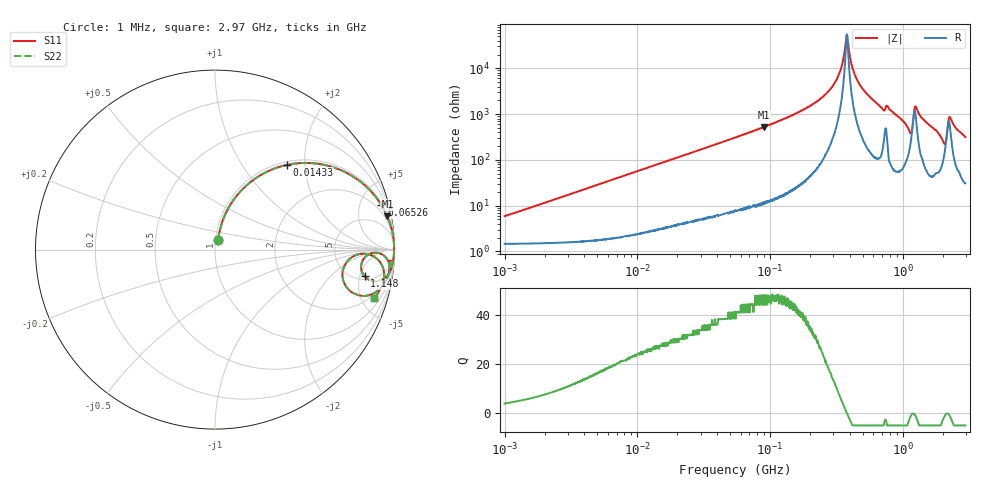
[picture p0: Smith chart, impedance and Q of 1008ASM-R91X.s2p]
!s-Parameter Generated by FASTRON Sdn. Bhd.
!FASTRON P/N : 1008ASM-R91X
!Keysight Technologies: E4991B_MY54100416_A.01.15
!Date: Tue Nov 21 09:40:02 2023
!Version  :Rev00  Wed Nov 22 15:18:00 2023
!Data & Calibration Information:
!Freq  S11  S21  S12  S22
!PortZ  Port1:50+j0  Port2:50+j0
!When reading reference impedance value at option line is always used.
! Remarks : This data is being provided solely for informational purposes.
# Hz S dB R 50
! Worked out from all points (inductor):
!   1599 points, 1 MHz to 2.97 GHz, reference 50 ohm
!   read as one part in series: L = 911 nH near 1.036 MHz
!   highest Q = 47.7 at 89.44 MHz (marker M1), where L = 924 nH
!   self-resonance near 377.9 MHz
!   S11 on the Smith chart (normalised r, x): 1 MHz: 1.03, +0.11; 14.33 MHz: 1.06, +1.61; 65.26 MHz: 1.18, +7.41; 1.148 GHz: 5.69, -5.95; 2.97 GHz: 1.62, -6.28
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1000000  -24.70 72.4  -0.14 -3.2  -0.14 -3.2  -24.70 72.4
3804036  -13.60 73.6  -0.34 -12.0  -0.34 -12.0  -13.60 73.6
1.432659e7  -4.19 49.8  -2.34 -38.1  -2.34 -38.1  -4.19 49.8
1.439846e7  -4.16 49.6  -2.35 -38.2  -2.35 -38.2  -4.16 49.6
5.477226e7  -0.50 17.8  -10.30 -70.8  -10.30 -70.8  -0.50 17.8
6.525633e7  -0.36 15.0  -11.70 -73.6  -11.70 -73.6  -0.36 15.0
8.944052e7  -0.19 10.9  -14.50 -77.9  -14.50 -77.9  -0.19 10.9
2.073156e8  -0.03 3.6  -24.10 -84.7  -24.10 -84.7  -0.03 3.6
3.140564e8  -0.02 1.1  -34.50 -83.7  -34.50 -83.7  -0.02 1.1
3.453811e8  -0.02 0.5  -40.50 -78.9  -40.50 -78.9  -0.02 0.5
3.798301e8  -0.02 -0.0  -54.80 0.4  -54.80 0.4  -0.02 -0.0
4.240331e8  -0.02 -0.6  -39.10 79.3  -39.10 79.3  -0.02 -0.6
4.781416e8  -0.02 -1.3  -32.60 83.4  -32.60 83.4  -0.02 -1.3
7.028992e8  -0.10 -4.3  -22.40 78.9  -22.40 78.9  -0.10 -4.3
7.846996e8  -0.07 -4.2  -22.70 81.3  -22.70 81.3  -0.07 -4.2
1.147801e9  -1.45 -10.1  -13.00 41.7  -13.00 41.7  -1.45 -10.1
1.262285e9  -0.33 -3.3  -23.30 54.8  -23.30 54.8  -0.33 -3.3
1.76507e9  -0.41 -12.2  -13.50 71.5  -13.50 71.5  -0.41 -12.2
2.020405e9  -1.64 -17.6  -9.69 49.9  -9.69 49.9  -1.64 -17.6
2.167021e9  -1.80 -1.7  -14.50 7.2  -14.50 7.2  -1.80 -1.7
2.278218e9  -0.62 -5.1  -19.20 48.8  -19.20 48.8  -0.62 -5.1
2.970126e9  -0.65 -17.0  -10.60 67.4  -10.60 67.4  -0.65 -17.0
